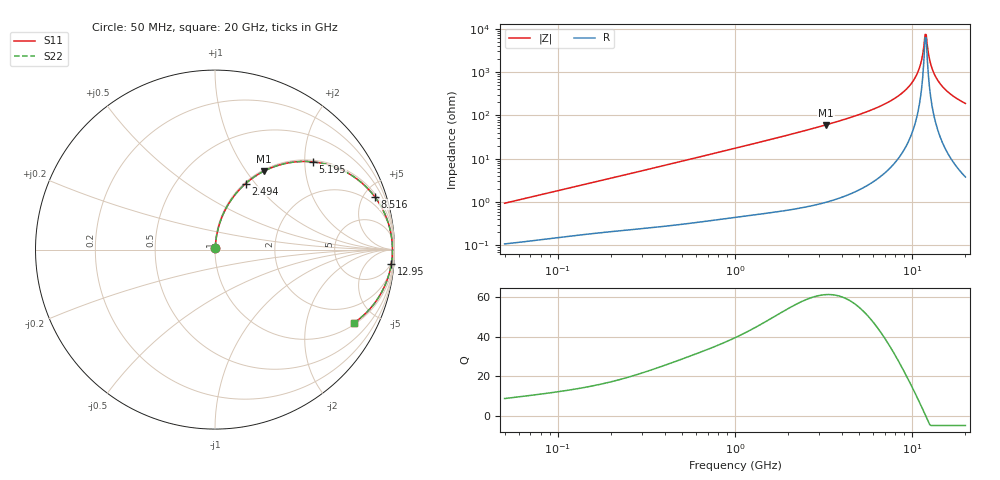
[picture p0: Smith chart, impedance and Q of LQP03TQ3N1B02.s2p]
!Murata Part Number: LQP03TQ3N1B02
!These Parameters are Measured in Series Mode Connection
!  o--[Z]--o
!Port1  Port2
!  o-------o
!Freq. Start=50[MHz] Stop=20[GHz], 401[Steps]
# Hz S RI R 50
!Freq.(Hz) S11(Real) S11(Imag) S21(Real) S21(Imag) S12(Real) S12(Imag) S22(Real) S22(Imag)
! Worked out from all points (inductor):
!   401 points, 50 MHz to 20 GHz, reference 50 ohm
!   read as one part in series: L = 2.94 nH near 51.52 MHz
!   highest Q = 61.3 at 3.265 GHz (marker M1), where L = 2.95 nH
!   self-resonance near 11.84 GHz
!   S11 on the Smith chart (normalised r, x): 50 MHz: 1.00, +0.02; 2.494 GHz: 1.02, +0.89; 5.195 GHz: 1.04, +2.19; 8.516 GHz: 1.22, +5.94; 12.95 GHz: 4, -24; 20 GHz: 1.08, -3.78
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5e7  0.00116 0.00929  0.9988 -0.00929  0.9988 -0.00929  0.00116 0.00929
1.364002e8  0.00235 0.0244  0.9977 -0.0244  0.9977 -0.0244  0.00235 0.0244
3.721004e8  0.00687 0.0646  0.9931 -0.0646  0.9931 -0.0646  0.00687 0.0646
1e9  0.0334 0.1675  0.9666 -0.1675  0.9666 -0.1675  0.0334 0.1675
2.493527e9  0.1708 0.3679  0.8292 -0.3679  0.8292 -0.3679  0.1708 0.3679
2.728004e9  0.1998 0.3916  0.8002 -0.3916  0.8002 -0.3916  0.1998 0.3916
3.265178e9  0.2711 0.4364  0.7289 -0.4364  0.7289 -0.4364  0.2711 0.4364
5.194772e9  0.5454 0.4887  0.4546 -0.4887  0.4546 -0.4887  0.5454 0.4887
7.442007e9  0.8062 0.3815  0.1938 -0.3815  0.1938 -0.3815  0.8062 0.3815
8.516016e9  0.8893 0.2954  0.1107 -0.2954  0.1107 -0.2954  0.8893 0.2954
9.600142e9  0.9456 0.2003  0.0544 -0.2003  0.0544 -0.2003  0.9456 0.2003
1.050288e10  0.9734 0.1203  0.0266 -0.1203  0.0266 -0.1203  0.9734 0.1203
1.115139e10  0.9843 0.0642  0.0157 -0.0642  0.0157 -0.0642  0.9843 0.0642
1.166392e10  0.9882 0.0214  0.0118 -0.0214  0.0118 -0.0214  0.9882 0.0214
1.183995e10  0.9886 0.00705  0.0114 -0.00705  0.0114 -0.00705  0.9886 0.00705
1.220001e10  0.9883 -0.0216  0.0117 0.0216  0.0117 0.0216  0.9883 -0.0216
1.257102e10  0.9862 -0.0503  0.0138 0.0503  0.0138 0.0503  0.9862 -0.0503
1.295331e10  0.9826 -0.0787  0.0174 0.0787  0.0174 0.0787  0.9826 -0.0787
1.375312e10  0.9704 -0.1344  0.0296 0.1344  0.0296 0.1344  0.9704 -0.1344
1.504638e10  0.9406 -0.2137  0.0594 0.2137  0.0594 0.2137  0.9406 -0.2137
1.721783e10  0.8736 -0.318  0.1264 0.318  0.1264 0.318  0.8736 -0.318
2e10  0.7764 -0.4068  0.2236 0.4068  0.2236 0.4068  0.7764 -0.4068
